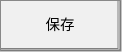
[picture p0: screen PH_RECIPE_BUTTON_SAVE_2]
VISUALIZATION PH_RECIPE_BUTTON_SAVE_2  // 122x52
VAR_IN_OUT
	RECIPE_CTRL_V2 : ST_RecipeCtrl_2;
END_VAR
    Button (0,0 120x50), "保存", input disabled if: (RECIPE_CTRL_V2.sStatus.bBusy) <> 0, text list: 'TextList_Recipe', text index: 112
        p55702900: SEL(RECIPE_CTRL_V2.sCmd.bRecipeSave, 16#000000, 16#00FF00)
        tap RECIPE_CTRL_V2.sCmd.bRecipeSave
END_VISUALIZATION
